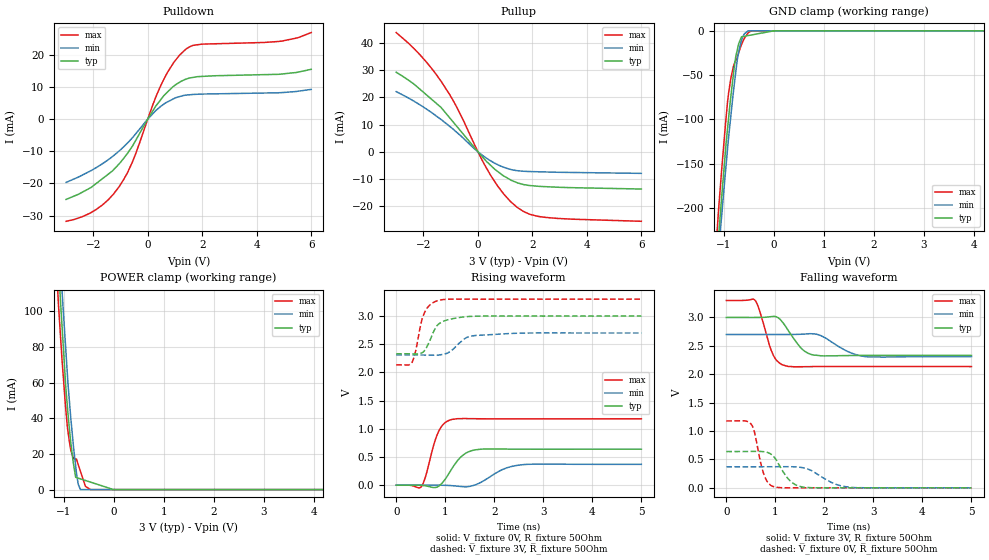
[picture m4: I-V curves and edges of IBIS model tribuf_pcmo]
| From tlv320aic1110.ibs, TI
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|   tribuf_pcmo Model
[Model]   tribuf_pcmo
Model_type   3-state
Polarity   Non-Inverting
Enable   Active-Low
Vmeas = 1.5
Vref = 1.5
Cref = 15pF
Rref = 50
|   typ   min   max
|   (nom PVT)   (Fast PVT)   (slow PVT)
|Average
C_comp   2.569e-12   2.559e-12   2.570e-12
|ON state : BUFFER OUTPUT TURNED HIGH
|C_comp (ON state)   2.570e-12   2.559e-12   2.569e-12
|OFF state: BUFFER IN HIGH IMPEDANCE
|C_comp (OFF state)   2.433e-12   2.431e-12   2.427e-12
| Where nom  PVT is Nominal Process,  3V,  65C
|   Fast PVT is Strong Process,   3.3V,  -40C
[Voltage Range]   3   2.7   3.3
|Ambient Temperature   25   105   -40
|Junction Temperature
[Temperature Range]   65   125   -40
[Pullup Reference]   3   2.7   3.3
[Pulldown Reference]   0   0   0
[Power Clamp Reference]   3   2.7   3.3
[GND Clamp Reference]   0   0   0
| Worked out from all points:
|   slope of the pulldown table from 0 to 0.45 V, typ, clamps not added: 78.7 ohm
|   slope of the pullup table from 0 to 0.45 V, typ, clamps not added: 93.2 ohm
|   falling waveform, V_fixture 3V, R_fixture 50Ohm: 20-80 % time 329ps typ, 457ps min, 245ps max; typ from 3 V to 2.33 V
|   rising waveform, V_fixture 0V, R_fixture 50Ohm: 20-80 % time 316ps typ, 445ps min, 235ps max; typ from 0 V to 0.639 V
|   rising waveform, V_fixture 3V, R_fixture 50Ohm: 20-80 % time 245ps typ, 319ps min, 188ps max; typ from 2.33 V to 3 V
|   falling waveform, V_fixture 0V, R_fixture 50Ohm: 20-80 % time 293ps typ, 449ps min, 183ps max; typ from 0.639 V to 0 V
[Pulldown]
|   Voltage   I(typ)   I(min)   I(max)
-3V       -24.97mA   -19.69mA   -31.76mA
-1.901V   -20.08mA   -15.14mA   -28.13mA
-1.459V   -17.18mA   -12.7mA    -25.13mA
-1.066V   -14.07mA   -10.03mA   -21.18mA
-564.6mV  -8.437mA   -5.831mA   -13.36mA
184.5mV   2.52mA     1.641mA    4.413mA
537.6mV   6.669mA    4.301mA    11.45mA
956.7mV   10.21mA    6.315mA    17.58mA
1.389V    12.34mA    7.392mA    21.61mA
1.986V    13.21mA    7.733mA    23.23mA
4.93V     13.96mA    8.187mA    24.19mA
6V        15.42mA    9.185mA    26.82mA
[GND Clamp]
|   Voltage   I(typ)   I(min)   I(max)
-3V       -1.784A    -1.712A    -1.878A
-1.134V   -248.8mA   -266.3mA   -221.8mA
-1.097V   -222.1mA   -240.7mA   -191.9mA
-1.046V   -186.5mA   -207.7mA   -155.8mA
-930.9mV  -110.6mA   -133.6mA   -80.44mA
-864.9mV  -74.37mA   -96.44mA   -53.9mA
-780mV    -34.07mA   -53.25mA   -34.98mA
-734.7mV  -21.37mA   -32.48mA   -29.67mA
-656.4mV  -7.484mA   -11.81mA   -16.23mA
-518.4mV  -5.352mA   0A         -2.34mA
-3.6mV    0A         0A         0A
6V        0A         0A         0A
[Pullup]
|   Voltage   I(typ)   I(min)   I(max)
-3V       29.24mA    22.11mA    43.82mA
-2.122V   22.93mA    17.21mA    35.59mA
-1.726V   19.51mA    14.6mA     30.96mA
-1.36V    16.35mA    11.92mA    26.03mA
-765.9mV  9.228mA    7.051mA    16.18mA
42.6mV    -485.9uA   -335.7uA   -865.6uA
451.8mV   -4.847mA   -3.238mA   -8.403mA
946.8mV   -8.884mA   -5.676mA   -15.52mA
1.435V    -11.35mA   -6.929mA   -20.37mA
1.891V    -12.39mA   -7.259mA   -22.92mA
2.488V    -12.82mA   -7.416mA   -24.12mA
6V        -13.69mA   -7.935mA   -25.55mA
[POWER Clamp]
|   Voltage   I(typ)   I(min)   I(max)
-3V       1.22A      1.173A     1.337A
-1.155V   148.4mA    167.5mA    129.8mA
-1.113V   127.7mA    146.9mA    106.6mA
-1.062V   103.6mA    123.6mA    84.03mA
-1.036V   92.02mA    112mA      72.98mA
-927.6mV  46.26mA    64.19mA    34.75mA
-858mV    25.77mA    39.44mA    21.9mA
-762mV    6.883mA    13.02mA    17.16mA
-667.2mV  6.023mA    0A         10.25mA
-462.3mV  4.165mA    0A         0A
-3.6mV    0A         0A         0A
6V        0A         0A         0A
[Ramp]
R_load = 50
|   typ   min   max
dV/dt_r   0.383231/3.1638e-10   0.222058/4.4425e-10   0.706803/2.34573e-10
dV/dt_f   0.40127/3.28822e-10   0.234028/4.56661e-10   0.699154/2.45069e-10
[Falling Waveform]
V_fixture = 3V
V_fixture_min = 2.7V
V_fixture_max = 3.3V
R_fixture = 50Ohm
|   Time   V(typ)   V(min)   V(max)
0s        3V         2.7V       3.3V
575ps     3V         2.7V       3.311V
675ps     3V         2.7V       3.126V
950ps     3.018V     2.7V       2.35V
1.075ns   2.983V     2.7V       2.204V
1.225ns   2.822V     2.7V       2.144V
1.525ns   2.459V     2.704V     2.132V
1.8ns     2.336V     2.709V     2.135V
2.825ns   2.331V     2.312V     2.136V
5ns       2.331V     2.31V      2.135V
[Rising Waveform]
V_fixture = 0V
V_fixture_min = 0V
V_fixture_max = 0V
R_fixture = 50Ohm
|   Time   V(typ)   V(min)   V(max)
0s        2.028nV    14.33nV    1.005nV
525ps     -3.151mV   91.61uV    -11.55mV
850ps     -26.38mV   128uV      924.2mV
975ps     78.76mV    -1.636mV   1.092V
1.125ns   278.1mV    -7.531mV   1.164V
1.375ns   541.7mV    -27.23mV   1.182V
1.7ns     636.2mV    39.11mV    1.178V
2.175ns   641.2mV    280.2mV    1.177V
2.55ns    638.8mV    361.3mV    1.177V
5ns       638.7mV    370.1mV    1.178V
[Rising Waveform]
V_fixture = 3V
V_fixture_min = 2.7V
V_fixture_max = 3.3V
R_fixture = 50Ohm
|   Time   V(typ)   V(min)   V(max)
0s        2.331V     2.31V      2.135V
325ps     2.329V     2.31V      2.18V
400ps     2.327V     2.31V      2.394V
525ps     2.35V      2.309V     2.939V
575ps     2.385V     2.309V     3.057V
850ps     2.847V     2.307V     3.275V
1.05ns    2.934V     2.345V     3.298V
1.4ns     2.987V     2.601V     3.3V
1.625ns   2.998V     2.657V     3.3V
5ns       3V         2.7V       3.3V
[Falling Waveform]
V_fixture = 0V
V_fixture_min = 0V
V_fixture_max = 0V
R_fixture = 50Ohm
|   Time   V(typ)   V(min)   V(max)
0s        638.8mV    370.2mV    1.178V
500ps     640.5mV    370.1mV    1.129V
575ps     641.3mV    370.2mV    977.7mV
700ps     640.2mV    370.4mV    441.9mV
775ps     634.7mV    370.6mV    216.4mV
950ps     564.1mV    371.2mV    24.14mV
1.275ns   145.8mV    372.1mV    -162.9uV
1.575ns   10.54mV    351.2mV    655.2uV
2.5ns     47.16uV    12.66mV    844uV
5ns       95.67uV    52.2uV     120.7uV
